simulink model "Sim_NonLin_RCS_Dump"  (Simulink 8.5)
settings: Solver=ode45  StartTime=0.0  StopTime=1250  FixedStep=Ts  RelTol=1e-3
InitFcn:
  | start1
StopFcn:
  | Pl
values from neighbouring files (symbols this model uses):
  com_dir = com_dir/sqrt(com_dir'*com_dir)    [start.m]    (also in start1.m; start2.m; start3.m)
  d2r = pi/180    (= 0.0174532925199)    [start.m]    (also in start1.m; start2.m; start3.m; Dead_Band_DF.m)
  ini = [wbo; atto; Hco]    [start.m]    (also in start1.m; start2.m; start3.m)
  KshR = 2*Wdot_Lim_RCS/WlimR    [start.m]    (also in start1.m; start2.m; start3.m)
  nt = 12    [start.m]    (also in start1.m; start2.m; start3.m)
  r2d = 180/pi    (= 57.2957795131)    [start.m]    (also in start1.m; start2.m; start3.m)
  thecmd = 20    [start.m]    (also in start1.m = 0.1; start2.m; start3.m)
  Wdot_Lim_RCS = 0.02*d2r    (= 0.000349065850399)    [start.m]    (also in start1.m; start2.m; start3.m)
  Wlim_RCS = 0.6*d2r    (= 0.010471975512)    [start.m]    (also in start1.m; start2.m; start3.m)
  wo = 0.0011    [start.m]    (also in start1.m; start2.m; start3.m)
undefined symbols (not defined in the file or in its folder): Mom_Dump, Phase_Plane, Rigbod_Dynam_LVLH, Wlim

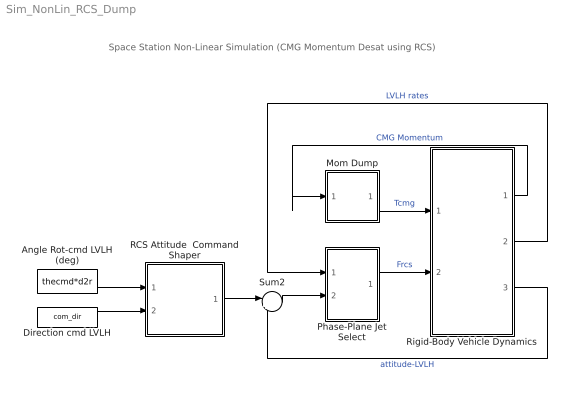
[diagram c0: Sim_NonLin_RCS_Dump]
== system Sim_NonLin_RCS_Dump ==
  note: Space Station Non-Linear Simulation (CMG Momentum Desat using RCS)
  Angle Rot-cmd LVLH (deg) : Constant  Value=thecmd*d2r
  Direction cmd LVLH : Constant  Value=com_dir
  Mom Dump : Subsystem
  Phase-Plane Jet Select : Subsystem
  RCS Attitude  Command Shaper : Subsystem
  Rigid-Body Vehicle Dynamics : Subsystem
  Sum2 : Sum  Inputs=|+-
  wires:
  Rigid-Body Vehicle Dynamics/3(atti-lv) -> Sum2/2  "attitude-LVLH"
  Rigid-Body Vehicle Dynamics/1(Hcmg) -> Mom Dump/1(Hcmg)  "CMG Momentum"
  Sum2/1 -> Phase-Plane Jet Select/2(atter)
  Rigid-Body Vehicle Dynamics/2(w-lv) -> Phase-Plane Jet Select/1(rater)  "LVLH rates"
  Direction cmd LVLH/1 -> RCS Attitude  Command Shaper/2(dir)
  Angle Rot-cmd LVLH (deg)/1 -> RCS Attitude  Command Shaper/1(cmd)
  Phase-Plane Jet Select/1(f(i)) -> Rigid-Body Vehicle Dynamics/2(f(i))  "Frcs"
  RCS Attitude  Command Shaper/1(att-cmd) -> Sum2/1
  Mom Dump/1(Tq) -> Rigid-Body Vehicle Dynamics/1(Tc)  "Tcmg"

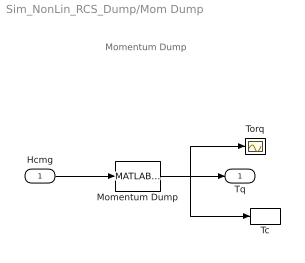
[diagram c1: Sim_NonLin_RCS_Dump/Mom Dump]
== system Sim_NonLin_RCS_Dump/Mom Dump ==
  note: Momentum Dump
  Hcmg : Inport  PortDimensions=3
  Momentum Dump : MATLABFcn  MATLABFcn=Mom_Dump( u(1:3) )  OutputDimensions=3
  Tc : ToWorkspace  VariableName=Tcmg  SampleTime=-1
  Torq : Scope
  Tq : Outport
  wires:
  Momentum Dump/1 -> Tc/1, Torq/1, Tq/1
  Hcmg/1 -> Momentum Dump/1

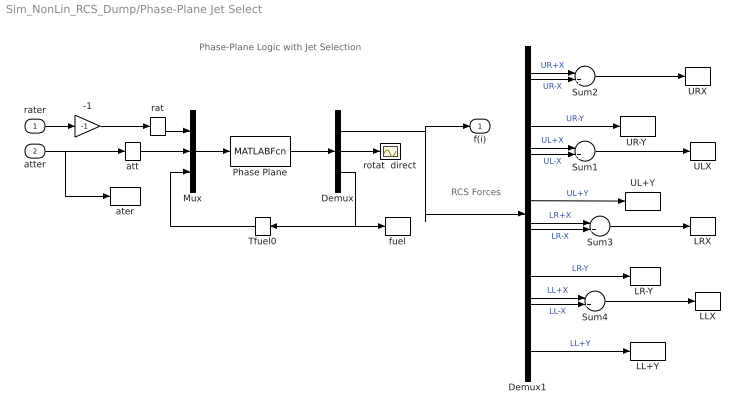
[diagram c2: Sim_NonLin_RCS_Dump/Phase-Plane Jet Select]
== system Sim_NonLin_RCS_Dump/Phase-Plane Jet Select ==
  note: RCS Forces
  note: Phase-Plane Logic with Jet Selection
  rater : Inport
  atter : Inport  Port=2
  -1 : Gain  Gain=-1
  Demux : Demux  Outputs=[nt, 3,1]
  Demux1 : Demux  Outputs=nt
  LL+Y : ToWorkspace  VariableName=LLPY  SampleTime=-1
  LLX : ToWorkspace  VariableName=LLX  SampleTime=-1
  "LR-Y " : ToWorkspace  VariableName=LRNY  SampleTime=-1
  LRX : ToWorkspace  VariableName=LRX  SampleTime=-1
  Mux : Mux  Inputs="[3  3  1]"
  Phase Plane : MATLABFcn  MATLABFcn=Phase_Plane( u(1:3), u(4:6), u(7) )  OutputDimensions=nt + 4
  Sum{1..4} (4 alike) : Sum  Inputs=|++
  Tfuel0 : Memory
  UL+Y : ToWorkspace  VariableName=ULPY  SampleTime=-1
  ULX : ToWorkspace  VariableName=ULX  SampleTime=-1
  "UR-Y " : ToWorkspace  VariableName=URNY  SampleTime=-1
  URX : ToWorkspace  VariableName=URX  SampleTime=-1
  ater : ToWorkspace  VariableName=atter  SampleTime=-1
  att : Memory
  fuel : ToWorkspace  VariableName=Fuel  SampleTime=-1
  rat : Memory
  rotat  direct : Scope
  f(i) : Outport
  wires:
  -1/1 -> rat/1
  Demux1/9 -> "LR-Y "/1  "LR-Y"
  Demux1/12 -> LL+Y/1  "LL+Y"
  Demux1/6 -> UL+Y/1  "UL+Y"
  Demux1/3 -> "UR-Y "/1  "UR-Y"
  Sum4/1 -> LLX/1
  Sum3/1 -> LRX/1
  Sum1/1 -> ULX/1
  Demux1/11 -> Sum4/2  "LL-X"
  Demux1/10 -> Sum4/1  "LL+X"
  Demux1/8 -> Sum3/2  "LR-X"
  Demux1/7 -> Sum3/1  "LR+X"
  Demux1/5 -> Sum1/2  "UL-X"
  Demux1/4 -> Sum1/1  "UL+X"
  Sum2/1 -> URX/1
  Demux1/2 -> Sum2/2  "UR-X"
  Demux1/1 -> Sum2/1  "UR+X"
  rat/1 -> Mux/1
  Mux/1 -> Phase Plane/1
  Phase Plane/1 -> Demux/1
  Tfuel0/1 -> Mux/3
  Demux/1 -> f(i)/1, Demux1/1
  Demux/2 -> rotat  direct/1
  rater/1 -> -1/1
  atter/1 -> ater/1, att/1
  att/1 -> Mux/2
  Demux/3 -> fuel/1, Tfuel0/1

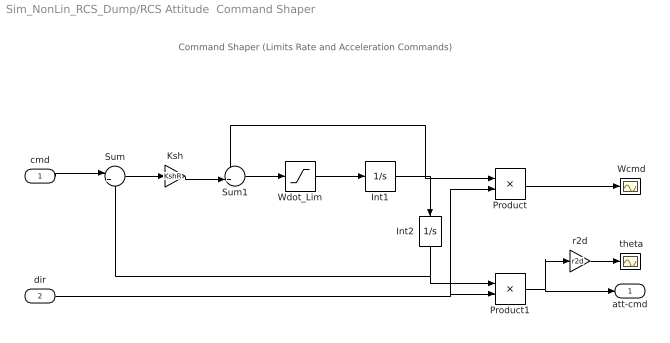
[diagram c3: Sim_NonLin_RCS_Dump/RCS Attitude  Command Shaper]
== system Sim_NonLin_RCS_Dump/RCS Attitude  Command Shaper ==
  note: Command Shaper (Limits Rate and Acceleration Commands)
  cmd : Inport  PortDimensions=1
  dir : Inport  Port=2  PortDimensions=3
  " Wcmd" : Scope
  " theta" : Scope
  Int1 : Integrator  LimitOutput=on  UpperSaturationLimit=Wlim_RCS  LowerSaturationLimit=-Wlim_RCS
  Int2 : Integrator  UpperSaturationLimit=Wlim  LowerSaturationLimit=-Wlim
  Ksh : Gain  Gain=KshR
  Product : Product
  Product1 : Product
  Sum : Sum  Inputs=|+-
  Sum1 : Sum  Inputs=-+|
  Wdot_Lim : Saturate  UpperLimit=Wdot_Lim_RCS  LowerLimit=-Wdot_Lim_RCS
  r2d : Gain  Gain=r2d
  att-cmd : Outport  PortDimensions=3
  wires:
  Wdot_Lim/1 -> Int1/1
  Sum1/1 -> Wdot_Lim/1
  Int1/1 -> Product/1, Sum1/1, Int2/1
  Sum/1 -> Ksh/1
  Ksh/1 -> Sum1/2
  Int2/1 -> Sum/2, Product1/1
  cmd/1 -> Sum/1
  dir/1 -> Product/2, Product1/2
  r2d/1 -> " theta"/1
  Product/1 -> " Wcmd"/1
  Product1/1 -> att-cmd/1, r2d/1

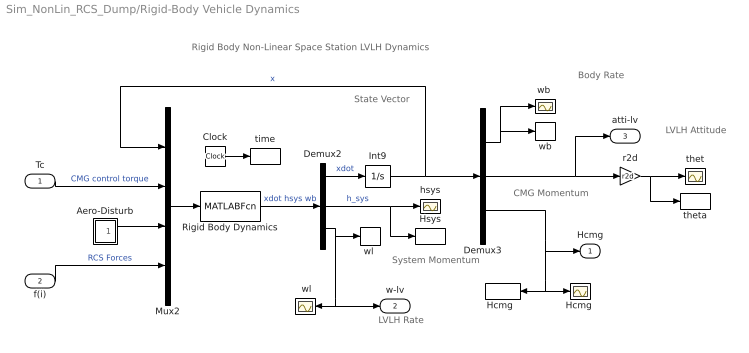
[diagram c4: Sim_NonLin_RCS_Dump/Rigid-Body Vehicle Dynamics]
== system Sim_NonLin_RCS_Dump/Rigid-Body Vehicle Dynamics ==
  note: Rigid Body Non-Linear Space Station LVLH Dynamics
  note: Body Rate
  note: LVLH Attitude
  note: CMG Momentum
  note: System Momentum
  note: LVLH Rate
  note: State Vector
  Tc : Inport  PortDimensions=3
  f(i) : Inport  Port=2  PortDimensions=nt
  " wl" : Scope
  Aero-Disturb : Subsystem
  Clock : Clock
  Demux2 : Demux  Outputs=[9,3,3]
  Demux3 : Demux  Outputs=[3,3,3]
  "Hcmg " : Scope
  "Hcmg  " : ToWorkspace  VariableName=Hcmg  SampleTime=-1
  Hsys : ToWorkspace  VariableName=Hsys  SampleTime=-1
  Int9 : Integrator  InitialCondition=ini
  Mux2 : Mux  Inputs=[9, 3, 3, nt]
  Rigid Body Dynamics : MATLABFcn  MATLABFcn=Rigbod_Dynam_LVLH( u(1:9), u(10:12), u(13:15), u(16:15+nt) )  OutputDimensions=15
  hsys : Scope
  r2d : Gain  Gain=r2d
  thet : Scope
  theta : ToWorkspace  VariableName=theta  SampleTime=-1
  time : ToWorkspace  VariableName=time  SampleTime=-1
  wb : ToWorkspace  VariableName=wb  SampleTime=-1
  "wb " : Scope
  "wl " : ToWorkspace  VariableName=wl  SampleTime=-1
  Hcmg : Outport
  w-lv : Outport  Port=2
  atti-lv : Outport  Port=3
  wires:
  Demux3/1 -> wb/1, "wb "/1
  Mux2/1 -> Rigid Body Dynamics/1
  Clock/1 -> time/1
  r2d/1 -> theta/1, thet/1
  f(i)/1 -> Mux2/4  "RCS Forces"
  Demux3/3 -> "Hcmg "/1, "Hcmg  "/1, Hcmg/1
  Demux3/2 -> atti-lv/1, r2d/1
  Demux2/2 -> Hsys/1, hsys/1  "h_sys"
  Demux2/3 -> " wl"/1, w-lv/1, "wl "/1
  Tc/1 -> Mux2/2  "CMG control torque"
  Int9/1 -> Mux2/1, Demux3/1  "x"
  Demux2/1 -> Int9/1  "xdot"
  Rigid Body Dynamics/1 -> Demux2/1  "xdot hsys wb"
  Aero-Disturb/1(Td) -> Mux2/3

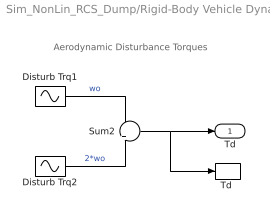
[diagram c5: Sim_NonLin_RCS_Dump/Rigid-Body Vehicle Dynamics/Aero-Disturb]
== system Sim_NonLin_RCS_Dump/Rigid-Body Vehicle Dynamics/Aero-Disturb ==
  note: Aerodynamic Disturbance Torques
  Disturb Trq1 : Sin  Amplitude=[1, 3, 1]  Bias="[1  8  1]"  Frequency=[wo, wo, wo]  SampleTime=0
  Disturb Trq2 : Sin  Amplitude=[1, 1, 1]*0.5  Frequency=[wo, wo, wo]*2  SampleTime=0
  Sum2 : Sum  Inputs=+|+
  "Td " : ToWorkspace  VariableName=Td  SampleTime=-1
  Td : Outport
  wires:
  Disturb Trq2/1 -> Sum2/2  "2*wo"
  Sum2/1 -> "Td "/1, Td/1
  Disturb Trq1/1 -> Sum2/1  "wo"
